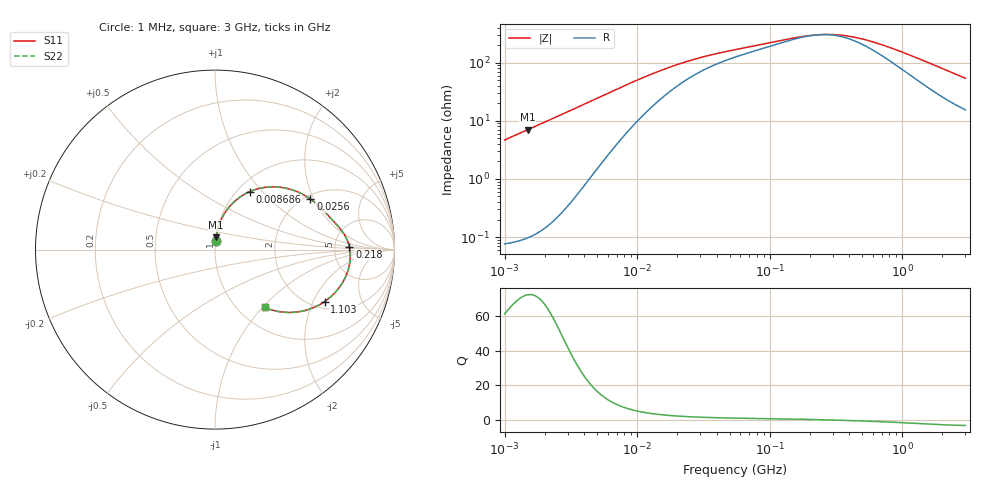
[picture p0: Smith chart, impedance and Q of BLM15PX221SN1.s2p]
! BLM15PX221SN1
# Hz S RI R 50
!Freq.(Hz) S11(Real) S11(Imag) S21(Real) S21(Imag) S12(Real) S12(Imag) S22(Real) S22(Imag)
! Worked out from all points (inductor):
!   401 points, 1 MHz to 3 GHz, reference 50 ohm
!   read as one part in series: L = 745 nH near 1.041 MHz
!   highest Q = 72.4 at 1.492 MHz (marker M1), where L = 746 nH
!   self-resonance near 239.1 MHz
!   S11 on the Smith chart (normalised r, x): 1 MHz: 1.00, +0.09; 8.686 MHz: 1.14, +0.86; 25.6 MHz: 2.14, +1.89; 218 MHz: 6.94, +0.45; 1.103 GHz: 2.30, -2.46; 3 GHz: 1.31, -1.03
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1000000  0.00293 0.0465  0.9971 -0.0465  0.9971 -0.0465  0.00293 0.0465
1492300  0.00582 0.0695  0.9942 -0.0695  0.9942 -0.0695  0.00582 0.0695
2461366  0.0155 0.1147  0.9845 -0.1147  0.9845 -0.1147  0.0155 0.1147
3823119  0.039 0.1762  0.961 -0.1762  0.961 -0.1762  0.039 0.1762
5820586  0.0939 0.2539  0.9061 -0.2539  0.9061 -0.2539  0.0939 0.2539
8686058  0.1945 0.3234  0.8055 -0.3234  0.8055 -0.3234  0.1945 0.3234
1.126754e7  0.2822 0.3474  0.7178 -0.3474  0.7178 -0.3474  0.2822 0.3474
1.461624e7  0.374 0.3462  0.626 -0.3462  0.626 -0.3462  0.374 0.3462
2.559965e7  0.5319 0.2812  0.4681 -0.2812  0.4681 -0.2812  0.5319 0.2812
3.597591e7  0.5917 0.2308  0.4083 -0.2308  0.4083 -0.2308  0.5917 0.2308
5.477226e7  0.6423 0.1776  0.3577 -0.1776  0.3577 -0.1776  0.6423 0.1776
1.219755e8  0.7155 0.0917  0.2845 -0.0917  0.2845 -0.0917  0.7155 0.0917
2.094008e8  0.7475 0.0201  0.2525 -0.0201  0.2525 -0.0201  0.7475 0.0201
2.179536e8  0.7489 0.0141  0.2511 -0.0141  0.2511 -0.0141  0.7489 0.0141
2.942768e8  0.754 -0.0332  0.246 0.0332  0.246 0.0332  0.754 -0.0332
3.894533e8  0.7496 -0.0818  0.2504 0.0818  0.2504 0.0818  0.7496 -0.0818
5.364635e8  0.7313 -0.1431  0.2687 0.1431  0.2687 0.1431  0.7313 -0.1431
8.005644e8  0.6805 -0.2263  0.3195 0.2263  0.3195 0.2263  0.6805 -0.2263
1.10276e9  0.6102 -0.29  0.3898 0.29  0.3898 0.29  0.6102 -0.29
1.818868e9  0.449 -0.3485  0.551 0.3485  0.551 0.3485  0.449 -0.3485
2.312676e9  0.3629 -0.3464  0.6371 0.3464  0.6371 0.3464  0.3629 -0.3464
3e9  0.2774 -0.3223  0.7226 0.3223  0.7226 0.3223  0.2774 -0.3223
